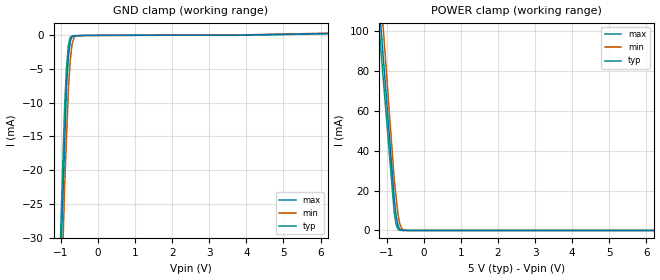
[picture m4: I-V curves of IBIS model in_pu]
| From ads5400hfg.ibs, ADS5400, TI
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[Model] in_pu
Model_type Input
Vinl = 800.000mV
Vinh = 2.00000V
C_comp 449.000fF 408.000fF 473.000fF
| variable typ   min   max
[Voltage Range] 5.00000V 4.75000V 5.25000V
[POWER Clamp Reference] 5.00000V 4.75000V 5.25000V
[GND Clamp Reference] 0.00000V 0.00000V 0.00000V
[Temperature Range] 25   85   -40
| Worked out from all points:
|   GND clamp passes 1 mA (typ) near -0.75 V on its own axis
|   POWER clamp passes 1 mA (typ) near -0.66 V on its own axis
[GND Clamp]
-5V       -696.2mA   -819.4mA   -722.2mA
-900mV    -16.14mA   -22.29mA   -10.58mA
-850mV    -7.849mA   -15.25mA   -4.827mA
-800mV    -3.284mA   -8.199mA   -1.513mA
-750mV    -945.3uA   -3.761mA   -333.4uA
-700mV    -230.4uA   -1.312mA   -97.93uA
-650mV    -85.69uA   -417.3uA   -88.91uA
-600mV    -77.66uA   -125.8uA   -79.89uA
-300mV    -33.29uA   -35.92uA   -34.28uA
3.8V      10.39uA    32.18uA    6.962uA
10V       619.8uA    705uA      591uA
[POWER Clamp]
-5V       1.024A     1.102A     961.3mA
-1.05V    76.36mA    89.98mA    65.95mA
-800mV    16.38mA    25.9mA     9.279mA
-750mV    7.749mA    17.24mA    3.174mA
-700mV    2.66mA     8.58mA     666.6uA
-650mV    614.7uA    3.451mA    132.6uA
-600mV    113.8uA    1.029mA    24.8uA
-550mV    21.29uA    238.8uA    21.89uA
-400mV    9.679uA    10.17uA    13.13uA
10V       0A         0A         0A
